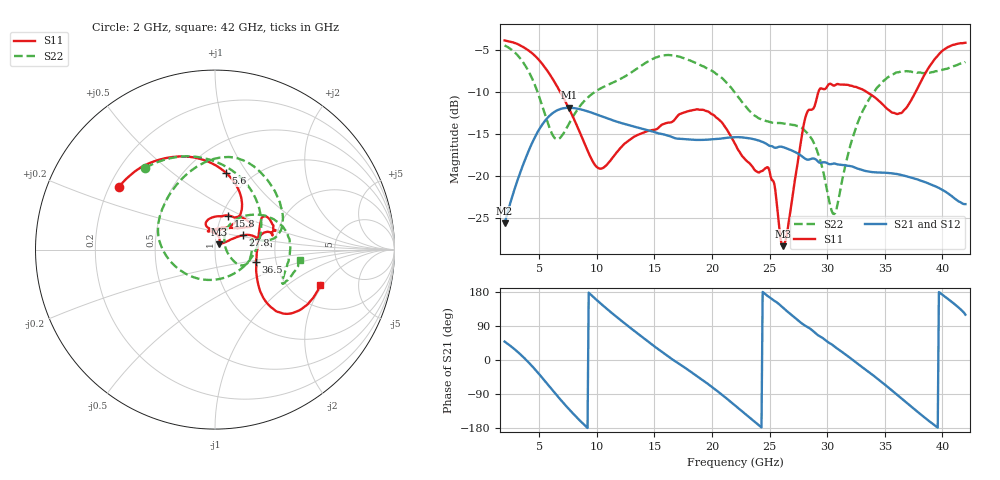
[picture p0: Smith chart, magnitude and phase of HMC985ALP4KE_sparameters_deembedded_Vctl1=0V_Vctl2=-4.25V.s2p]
!s2p File: Measurements: S11, S21, S12, S22
# GHz S dB R 50.0
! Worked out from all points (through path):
!   401 points, 2 GHz to 42 GHz, reference 50 ohm
!   highest |S21| = -11.89 dB at 7.6 GHz (marker M1); lowest = -25.7 dB at 2 GHz (marker M2)
!   lowest |S11| = -28.4 dB at 26.2 GHz (marker M3), VSWR 1.08, Z = 52.3 + j3.17 ohm
!   |S11| at or under -10 dB: 6.821 GHz to 29.25 GHz (22.43 GHz wide, 124 % of centre); 33.42 GHz to 37.69 GHz (4.27 GHz wide, 12 % of centre)
!   |S22| runs from -24.5 to -4.5 dB; largest |S21 - S12| = 0.00024
!   S11 on the Smith chart (normalised r, x): 2 GHz: 0.24, +0.28; 5.6 GHz: 0.76, +0.80; 15.8 GHz: 1.07, +0.42; 27.8 GHz: 1.34, +0.22; 36.5 GHz: 1.57, -0.23; 42 GHz: 2.95, -1.89
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2  -3.88 147.0  -25.66 48.6  -25.67 48.6  -4.47 130.5
3.6  -4.66 120.3  -18.70 8.3  -18.70 8.3  -6.48 84.9
4.7  -5.80 99.5  -15.21 -26.9  -15.22 -26.9  -9.43 43.3
5.6  -7.29 81.9  -13.29 -59.1  -13.30 -59.1  -13.07 -3.8
6.5  -9.22 66.5  -12.24 -92.0  -12.25 -92.1  -15.63 -69.2
7.6  -12.03 54.8  -11.89 -130.2  -11.90 -130.2  -13.76 -136.0
8.7  -15.38 55.0  -12.12 -164.8  -12.12 -164.8  -11.43 -170.3
10.4  -19.14 89.6  -12.89 147.4  -12.90 147.4  -9.54 162.3
15.4  -14.22 75.7  -14.97 27.3  -14.97 27.3  -5.79 86.9
15.8  -13.83 68.7  -15.06 18.4  -15.07 18.4  -5.66 81.8
19.4  -12.23 33.3  -15.71 -57.5  -15.71 -57.6  -7.07 34.7
22  -16.19 51.2  -15.40 -119.8  -15.40 -119.8  -10.10 9.9
24.9  -19.04 104.7  -16.35 167.5  -16.36 167.4  -13.54 13.2
26.2  -28.37 52.6  -16.60 137.1  -16.60 137.1  -13.77 -2.8
27.8  -15.23 27.2  -17.65 96.6  -17.65 96.5  -14.30 -24.9
28.7  -12.11 12.6  -17.95 78.4  -17.95 78.4  -15.69 -31.8
30.6  -9.26 19.5  -18.53 36.5  -18.53 36.5  -24.55 17.3
32.8  -9.59 34.0  -19.21 -13.4  -19.21 -13.4  -13.16 53.0
35.4  -12.22 11.7  -19.67 -74.7  -19.68 -74.7  -8.16 21.0
36.5  -12.47 -16.7  -19.91 -102.6  -19.92 -102.6  -7.56 7.0
39.5  -5.86 -43.7  -21.31 -176.1  -21.31 -176.2  -7.53 -26.3
42  -4.16 -18.6  -23.37 119.6  -23.38 119.5  -6.44 -7.0
